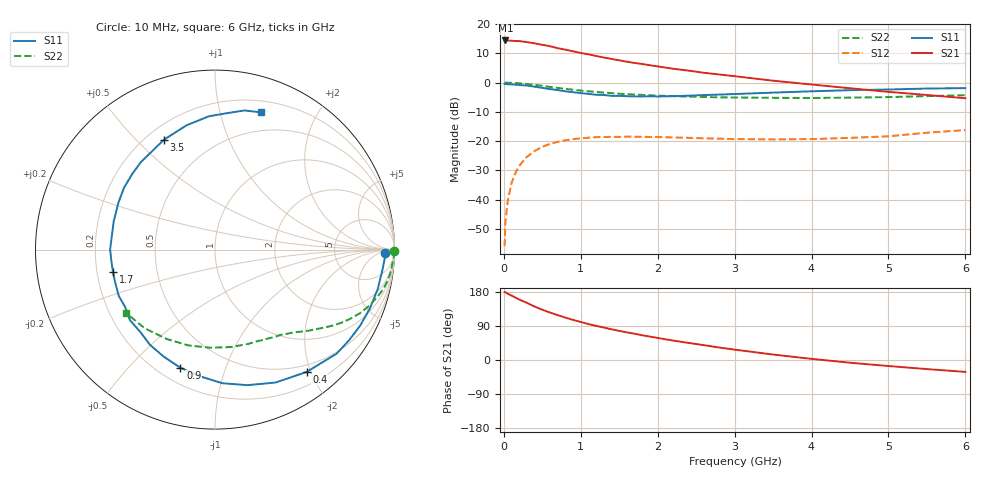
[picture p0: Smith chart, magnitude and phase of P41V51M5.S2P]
! SIEMENS Small Signal Semiconductors
! BFP182
! Si NPN RF Bipolar Junction Transistor in SOT143
! VCE = 1.5 V  IC = 1.5 mA
! Common Emitter S-Parameters:  March  1996
# GHz  S  MA  R  50
!  f  S11  S21  S12  S22
! GHz  MAG  ANG  MAG  ANG  MAG  ANG  MAG  ANG
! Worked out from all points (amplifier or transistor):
!   36 points, 10 MHz to 6 GHz, reference 50 ohm
!   highest |S21| = 14.4 dB at 20 MHz (marker M1)
!   |S21| within 3 dB of that: start of sweep to 770.1 MHz
!   unconditionally stable (mu >= 1): 2.355 GHz to end of sweep
!   at 250 MHz: K = 0.12, MSG = 20.4 dB, |S12| = -26.8 dB
!   at 1.4 GHz: K = 0.62, MSG = 13.3 dB, |S12| = -18.5 dB
!   at 6 GHz: K = 1.07, MAG = 3.8 dB, |S12| = -16.2 dB
!   S11 on the Smith chart (normalised r, x): 10 MHz: 30, -12; 400 MHz: 0.39, -1.93; 900 MHz: 0.29, -0.71; 1.7 GHz: 0.27, -0.10; 3.5 GHz: 0.27, +0.61; 6 GHz: 0.31, +1.34
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0.01  0.9448 -1.3  5.242 179.4  0.0016 86.0  0.9985 -0.5
0.02  0.9475 -2.8  5.262 178.6  0.0041 84.5  0.9992 -1.1
0.05  0.9394 -7.2  5.248 175.0  0.0094 85.6  0.9956 -2.7
0.1  0.933 -13.6  5.213 170.0  0.0192 82.2  0.9896 -5.4
0.15  0.9233 -20.7  5.146 164.9  0.0285 76.8  0.9837 -8.1
0.2  0.913 -27.7  5.134 159.8  0.0376 73.2  0.975 -10.7
0.25  0.9015 -34.2  5.034 155.0  0.0455 69.1  0.9621 -13.3
0.4  0.8514 -53.2  4.692 141.1  0.0678 58.9  0.9151 -20.0
0.5  0.8139 -65.5  4.433 132.6  0.0801 52.2  0.8809 -23.8
0.6  0.7764 -76.6  4.195 125.2  0.0898 46.4  0.8446 -27.3
0.7  0.7458 -86.8  3.88 118.3  0.0973 41.3  0.8122 -30.2
0.9  0.6862 -106.3  3.433 105.8  0.1085 32.7  0.7561 -34.8
1.1  0.6423 -124.4  3.047 94.8  0.1145 25.9  0.7098 -38.8
1.4  0.5938 -147.5  2.541 81.1  0.1185 17.8  0.6611 -43.8
1.7  0.582 -167.8  2.17 69.2  0.1188 12.6  0.625 -48.2
1.9  0.5844 180.0  1.983 61.7  0.1178 9.7  0.6071 -51.2
2.2  0.586 164.3  1.729 51.3  0.1156 6.8  0.5891 -55.8
2.8  0.6249 137.5  1.379 32.9  0.1103 4.7  0.5602 -66.2
3.5  0.6752 114.9  1.079 14.4  0.107 5.4  0.5501 -80.8
4.5  0.7436 92.6  0.802 -7.2  0.1137 10.9  0.5542 -105.6
5.5  0.7926 78.0  0.615 -24.0  0.1394 14.4  0.588 -131.9
6  0.8058 71.6  0.541 -31.4  0.1543 12.1  0.6089 -144.7
